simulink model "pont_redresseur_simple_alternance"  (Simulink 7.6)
settings: Solver=ode15s  StartTime=0.0  StopTime=0.1  RelTol=1e-3
StopFcn:
  | close all
  | load signaux.mat
  | plotyy(x(1,:),x(2,:),x(1,:),x(3,:))
  | grid
  | title('Redressement simple alternance')
  | gtext('Sans capacité')
  | gtext('Avec capacité')
  | xlabel('temps')
libraries: fl_lib x12, nesl_utility x4, elec_lib x1

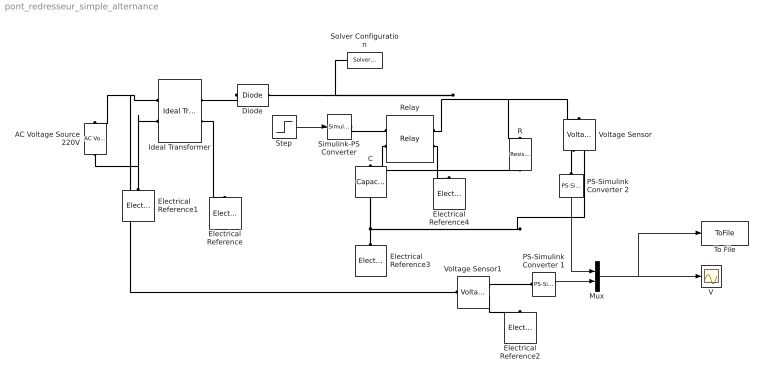
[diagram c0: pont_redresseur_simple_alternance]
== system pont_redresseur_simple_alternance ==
  AC Voltage Source 220V : fl_lib/Electrical/Electrical Sources/AC Voltage Source  DialogController=NetworkEngine.DynNeDlgSource  SystemSampleTime=-1  amp=220 V  shift=0 rad  omega=60 Hz  i_Log=off  v_Log=off  LocalVarNames=|i|v  LocalVarDescs=|i|v  LocalVarLogging=[0 0]
  C : fl_lib/Electrical/Electrical Elements/Capacitor  DialogController=NetworkEngine.DynNeDlgSource  SystemSampleTime=-1  c=1e-03 F  v0=0 V  r=1e-06 Ohm  g=0 1/Ohm  i_Log=off  v_Log=off  vc_Log=off  LocalVarNames=|i|v|vc  LocalVarDescs=|i|v|Internal variable for voltage across capacitor term  LocalVarLogging=[0 0 0]
  Diode : fl_lib/Electrical/Electrical Elements/Diode  DialogController=NetworkEngine.DynNeDlgSource  SystemSampleTime=-1  Vf=0.6 V  Ron=0.3 Ohm  Goff=1e-08 1/Ohm  i_Log=off  v_Log=off  LocalVarNames=|i|v  LocalVarDescs=|i|v  LocalVarLogging=[0 0]
  Electrical Reference{,1..4} (5 alike) : fl_lib/Electrical/Electrical Elements/Electrical Reference  DialogController=NetworkEngine.DynNeDlgSource  SystemSampleTime=-1  i_Log=off  LocalVarNames=|i  LocalVarDescs=|i  LocalVarLogging=0
  Ideal Transformer : fl_lib/Electrical/Electrical Elements/Ideal Transformer  DialogController=NetworkEngine.DynNeDlgSource  SystemSampleTime=-1  n=18  i1_Log=off  v1_Log=off  i2_Log=off  v2_Log=off  LocalVarNames=|i1|v1|i2|v2  LocalVarDescs=|i1|v1|i2|v2  LocalVarLogging=[0 0 0 0]
  Mux : Mux  Inputs=2
  PS-Simulink Converter 1 : nesl_utility/PS-Simulink Converter  DialogController=NetworkEngine.DynNeUtilDlgSource  SystemSampleTime=-1  PhysicalDomain=network_engine_domain  LeftPortType=input  RightPortType=output  SubClassName=ps_output  Unit=1  AffineConversion=off
  PS-Simulink Converter 2 : nesl_utility/PS-Simulink Converter  DialogController=NetworkEngine.DynNeUtilDlgSource  SystemSampleTime=-1  PhysicalDomain=network_engine_domain  LeftPortType=input  RightPortType=output  SubClassName=ps_output  Unit=1  AffineConversion=off
  R : fl_lib/Electrical/Electrical Elements/Resistor  Tag=Factory Generic  DialogController=NetworkEngine.DynNeDlgSource  SystemSampleTime=-1  R=20e3 Ohm  i_Log=off  v_Log=off  LocalVarNames=|current|voltage|power  LocalVarDescs=|Resistor current (A)|Voltage across resistor (V)|Power (W)  LocalVarLogging=[0 0 0]
  Relay : elec_lib/Passive Devices/Relay  DialogController=NetworkEngine.DynNeDlgSource  SystemSampleTime=-1  T_brk_C_S1=0 s  T_mak_C_S1=0 s  T_brk_C_S2=0 s  T_mak_C_S2=0 s  R_closed=0.01 Ohm  G_open=1e-08 1/Ohm  Threshold=0  initial_state=1  current_cs1_Log=off  current_cs2_Log=off  voltage_cs1_Log=off  voltage_cs2_Log=off  LocalVarNames=|current_cs1|current_cs2|voltage_cs1|voltage_cs2  LocalVarDescs=|Current flowing from C to S1 (A)|Current flowing from C to S2 (A)|Voltage across C - S1 (V)|Voltage across C - S2 (V)  LocalVarLogging=[0 0 0 0]
  Simulink-PS Converter : nesl_utility/Simulink-PS Converter  DialogController=NetworkEngine.DynNeUtilDlgSource  SystemSampleTime=-1  PhysicalDomain=network_engine_domain  LeftPortType=input  RightPortType=output  SubClassName=ps_input  Unit=1  AffineConversion=off  InputFilterTimeConstant=.001  UdotUserProvided=0
  Solver Configuration : nesl_utility/Solver Configuration  DialogController=NetworkEngine.DynNeUtilDlgSource  SystemSampleTime=-1  PhysicalDomain=network_engine_domain  LeftPortType=input  RightPortType=generic  SubClassName=solver  Accelerate=off  Profile=off  ResidualTolerance=1e-9  MaxNonlinIter=12  MaxModeIter=2  DoFixedCost=off  UseLocalSampling=off  DoDC=off  LinearAlgebra=Sparse  LocalSolverSampleTime=.001  LocalSolverChoice=NE_BACKWARD_EULER_ADVANCER  UseLocalSolver=off
  Step : Step  Time=0.05
  To File : ToFile  Filename=signaux  MatrixName=x
  V : Scope
  Voltage Sensor : fl_lib/Electrical/Electrical Sensors/Voltage Sensor  DialogController=NetworkEngine.DynNeDlgSource  SystemSampleTime=-1  i1_Log=off  v1_Log=off  LocalVarNames=|i1|v1  LocalVarDescs=|i1|v1  LocalVarLogging=[]
  Voltage Sensor1 : fl_lib/Electrical/Electrical Sensors/Voltage Sensor  DialogController=NetworkEngine.DynNeDlgSource  SystemSampleTime=-1  i1_Log=off  v1_Log=off  LocalVarNames=|i1|v1  LocalVarDescs=|i1|v1  LocalVarLogging=[]
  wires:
  PS-Simulink Converter 2/1 -> Mux/1
  PS-Simulink Converter 1/1 -> Mux/2
  Mux/1 -> To File/1, V/1
  Step/1 -> Simulink-PS Converter/1
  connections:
  PS-Simulink Converter 2/LConn1 -- Voltage Sensor/RConn1
  AC Voltage Source 220V/RConn1 -- Electrical Reference1/LConn1 -- Ideal Transformer/LConn2
  Voltage Sensor1/RConn1 -- PS-Simulink Converter 1/LConn1
  Voltage Sensor1/RConn2 -- Electrical Reference2/LConn1
  Voltage Sensor1/LConn1 -- Ideal Transformer/LConn1 -- AC Voltage Source 220V/LConn1
  Ideal Transformer/RConn2 -- Electrical Reference/LConn1
  Diode/LConn1 -- Ideal Transformer/RConn1
  Voltage Sensor/RConn2 -- R/RConn1 -- Electrical Reference3/LConn1 -- C/RConn1
  Relay/RConn1 -- Diode/RConn1 -- Solver Configuration/RConn1 -- Voltage Sensor/LConn1 -- R/LConn1
  Relay/LConn2 -- C/LConn1
  Simulink-PS Converter/RConn1 -- Relay/LConn1
  Relay/RConn2 -- Electrical Reference4/LConn1
